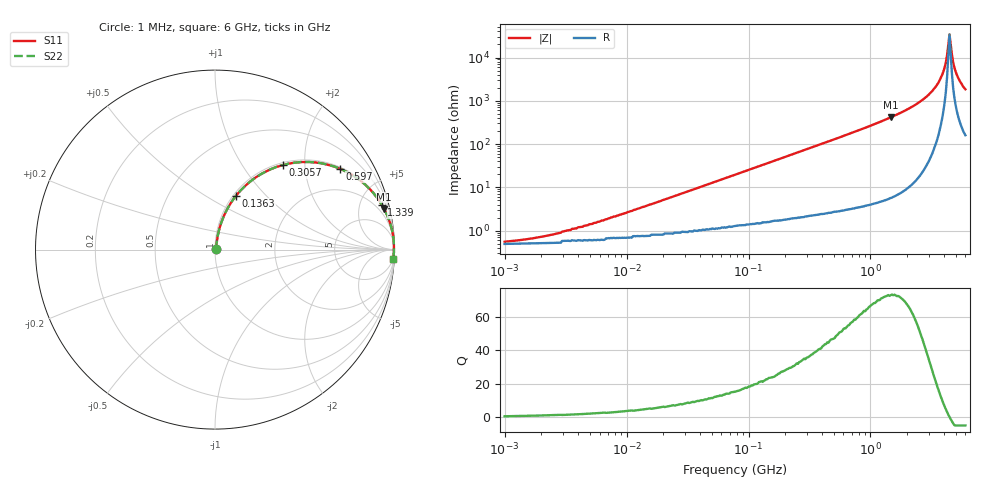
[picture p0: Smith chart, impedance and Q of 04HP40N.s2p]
# MHz S MA R 50
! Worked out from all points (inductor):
!   378 points, 1 MHz to 6 GHz, reference 50 ohm
!   read as one part in series: L = 40 nH near 8.165 MHz
!   highest Q = 73.2 at 1.468 GHz (marker M1), where L = 44.9 nH
!   self-resonance near 4.445 GHz
!   S11 on the Smith chart (normalised r, x): 1 MHz: 1.01, +0.01; 136.3 MHz: 1.03, +0.69; 305.7 MHz: 1.04, +1.54; 597 MHz: 1.06, +3.06; 1.339 GHz: 1.10, +7.40; 6 GHz: 4, -37
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1  0.005392 27.5  0.995 -0.1  0.995 -0.1  0.005392 27.5
1.953  0.007111 43.1  0.995 -0.3  0.995 -0.3  0.007111 43.1
4.279  0.012 60.8  0.994 -0.6  0.994 -0.6  0.012 60.8
18.312  0.046 77.4  0.991 -2.6  0.991 -2.6  0.046 77.4
78.359  0.191 75.3  0.969 -11.0  0.969 -11.0  0.191 75.3
136.334  0.32 68.8  0.933 -18.7  0.933 -18.7  0.32 68.8
305.747  0.603 51.3  0.781 -37.1  0.781 -37.1  0.603 51.3
335.312  0.638 48.8  0.753 -39.7  0.753 -39.7  0.638 48.8
597.02  0.83 32.9  0.543 -56.0  0.543 -56.0  0.83 32.9
1338.893  0.962 15.1  0.26 -74.1  0.26 -74.1  0.962 15.1
1434.864  0.967 13.9  0.24 -75.3  0.24 -75.3  0.967 13.9
1468.359  0.969 13.5  0.234 -75.7  0.234 -75.7  0.969 13.5
2554.767  0.993 5.9  0.104 -82.9  0.104 -82.9  0.993 5.9
3002.635  0.995 4.1  0.072 -84.2  0.072 -84.2  0.995 4.1
3529.019  0.997 2.4  0.042 -84.5  0.042 -84.5  0.997 2.4
4053.066  0.997 1.0  0.017 -80.2  0.017 -80.2  0.997 1.0
4244.504  0.997 0.5  0.008866 -71.5  0.008866 -71.5  0.997 0.5
4444.984  0.997 0.0  0.002927 -4.0  0.002927 -4.0  0.997 0.0
4654.933  0.997 -0.5  0.008604 68.3  0.008604 68.3  0.997 -0.5
4874.798  0.997 -0.9  0.017 77.5  0.017 77.5  0.997 -0.9
5346.175  0.996 -1.9  0.033 81.4  0.033 81.4  0.996 -1.9
6000  0.994 -3.1  0.054 81.9  0.054 81.9  0.994 -3.1
